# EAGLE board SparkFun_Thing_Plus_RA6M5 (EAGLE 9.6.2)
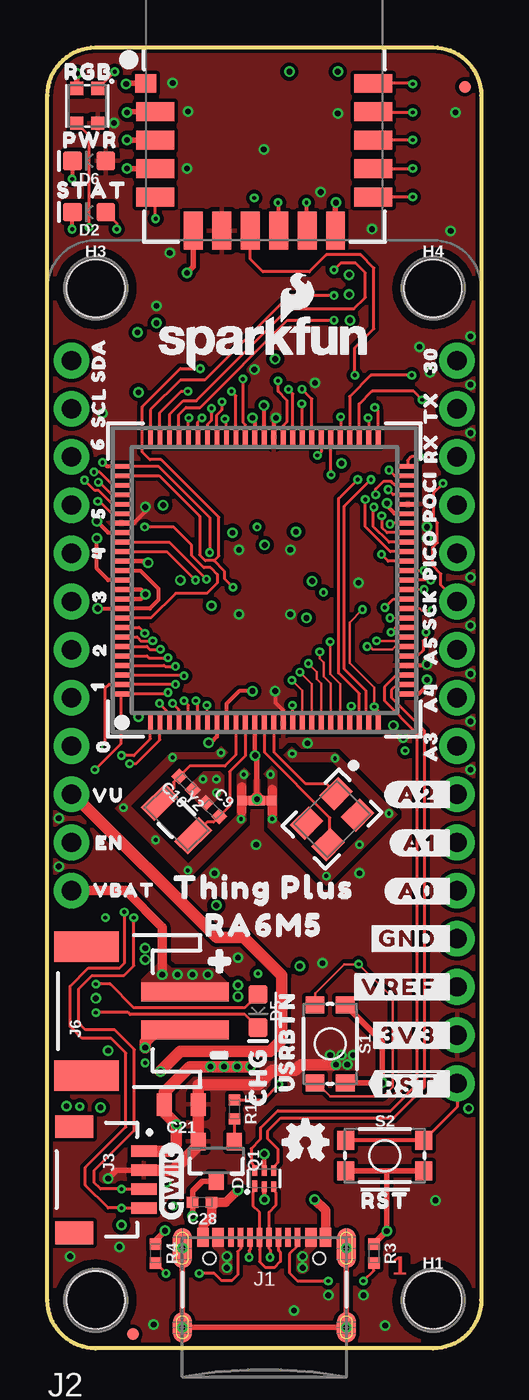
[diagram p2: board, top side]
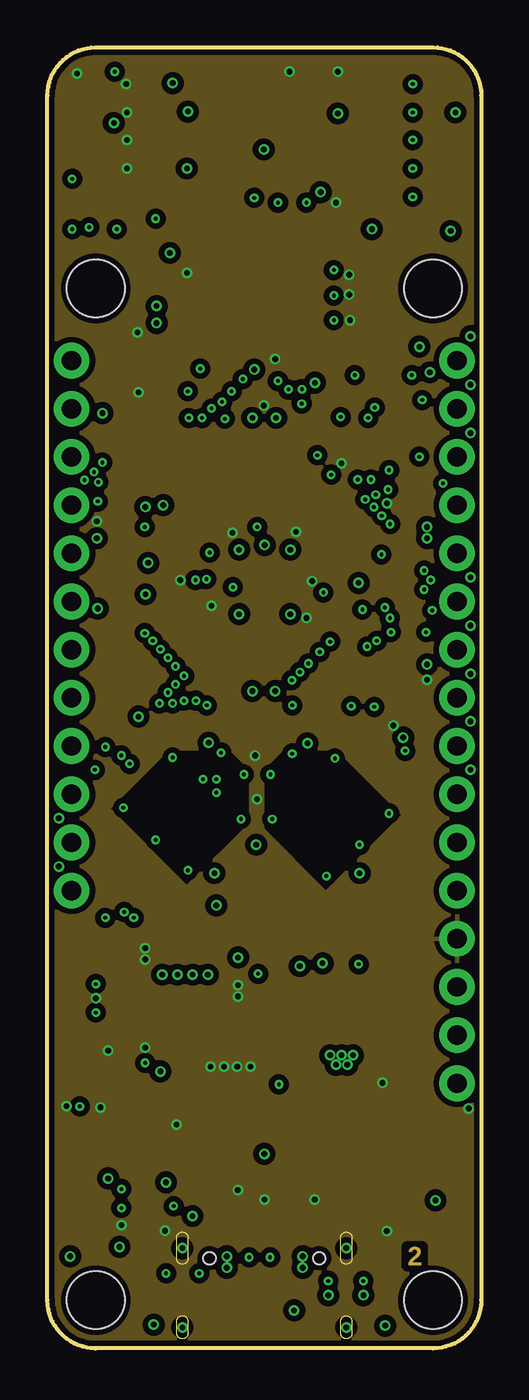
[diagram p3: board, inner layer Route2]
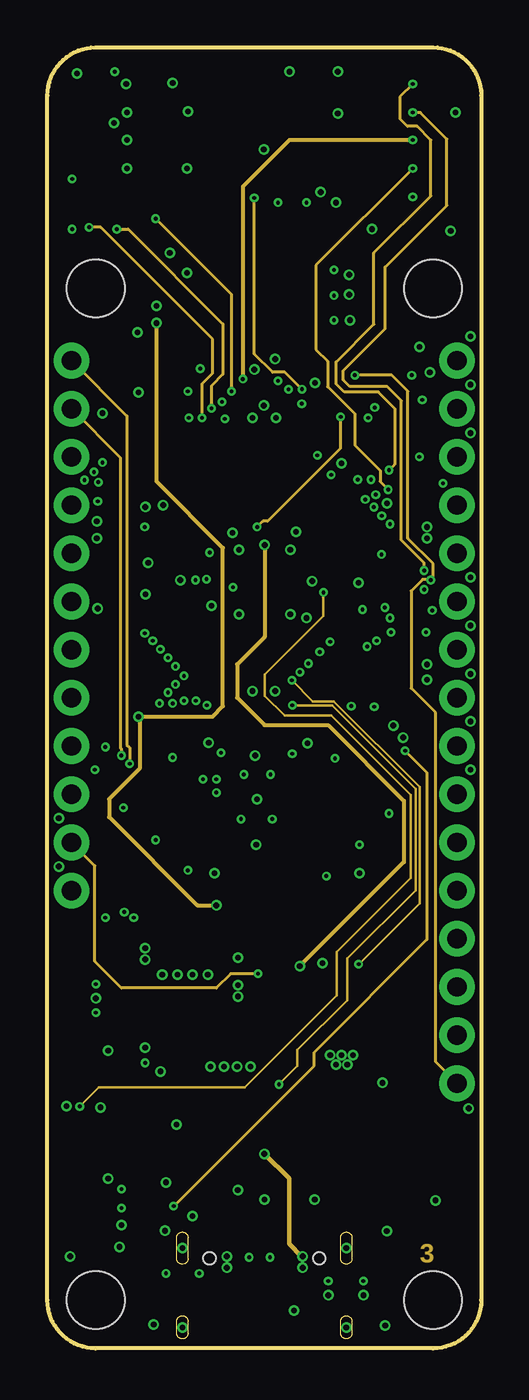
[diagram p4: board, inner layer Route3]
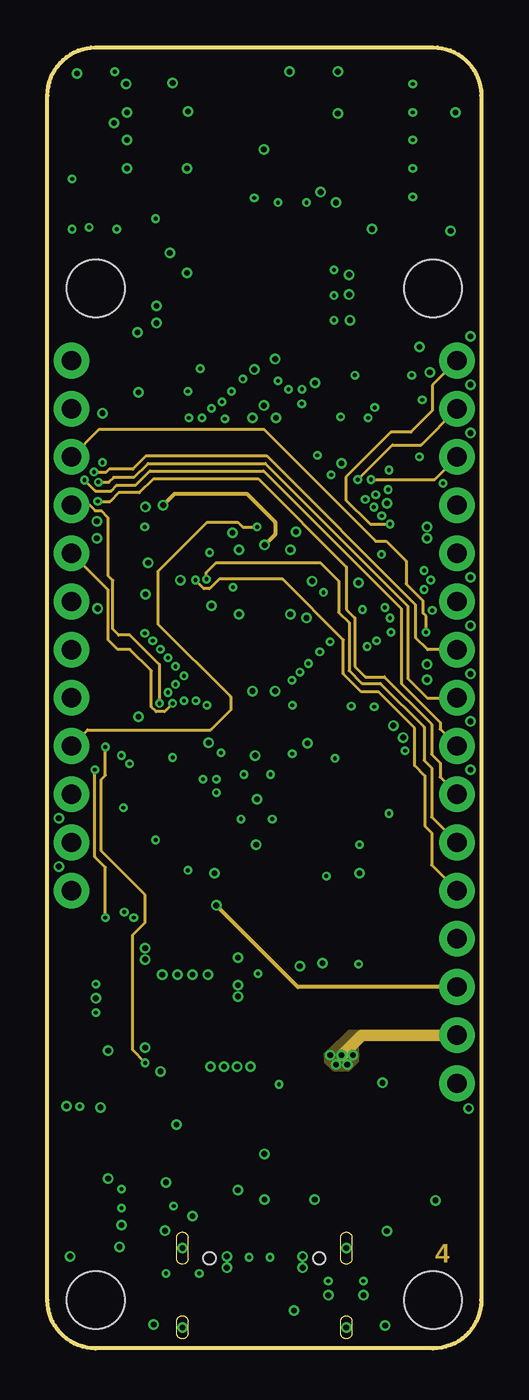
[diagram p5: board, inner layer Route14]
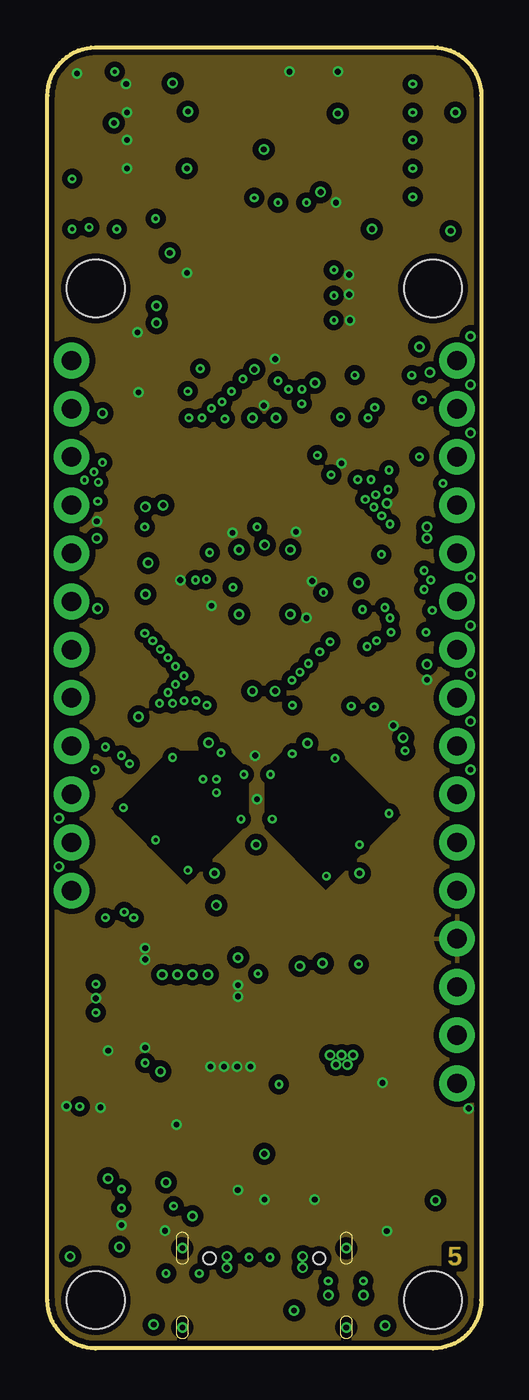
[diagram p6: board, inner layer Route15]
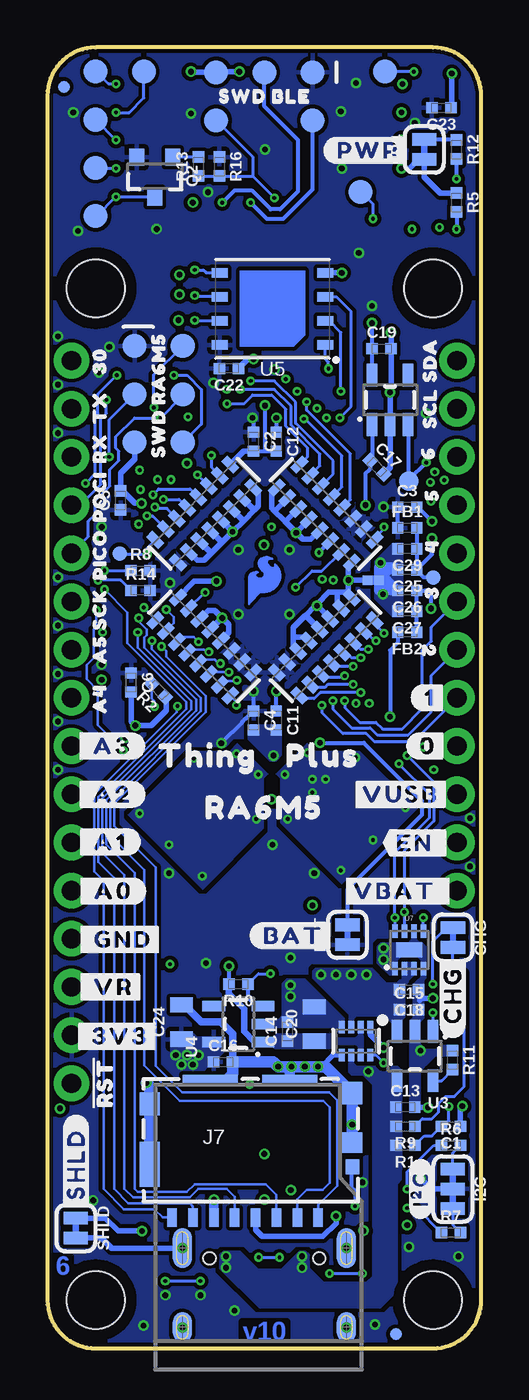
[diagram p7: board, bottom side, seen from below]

Size 22.86 x 68.58 mm. Coordinates in mm from the lower left corner, seen from the top.
Outline: 0,66.04 arc-90 2.54,68.58 20.32,68.58 arc-90 22.86,66.04 22.86,2.54 arc-90 20.32,0 2.54,0 arc-90 0,2.54 0,66.04
Copper layers (1+2*3+14*15+16): Top 0.035mm / dielectric 0.0994mm / Route2 0.0152mm / dielectric 0.55mm / Route3 0.0152mm / dielectric 0.1088mm / Route14 0.0152mm / dielectric 0.55mm / Route15 0.0152mm / dielectric 0.0994mm / Bottom 0.035mm
Design rules "SparkFun-6-Layer-Minimum-JLCPCB": minimum track width 0.09mm, minimum drill 0.2mm, track to track 0.09mm, track to pad 5mil, pad to pad 5mil, via to via 5mil, smd to smd 5mil, copper to edge 7mil, drill to drill 7mil, minimum pad ring 5mil, minimum via ring 5mil, stop-mask expansion 2.5mil, vias tented up to drill 25mil, thermal gap 10mil
Net classes: 2 CLK signals: width 0.15 mm, drill 0.2 mm, clearance 0.15 mm to class 0, clearance 0.15 mm to class 1, clearance 0.15 mm; 3 Analog Ground: width 0.2 mm, clearance 0.2 mm to class 1, clearance 0.3 mm to class 2; 4 Power: width 0.2 mm, drill 0.3 mm, clearance 0.2 mm to class 0, clearance 0.1 mm to class 1, clearance 0.15 mm to class 2, clearance 0.2 mm to class 3, clearance 0.2 mm; 5 USB diff: width 0.16 mm, drill 0.2 mm, clearance 0.3 mm to class 0, clearance 0.3 mm to class 1, clearance 0.3 mm to class 2, clearance 0.3 mm to class 3, clearance 0.2 mm to class 4, clearance 0.22 mm

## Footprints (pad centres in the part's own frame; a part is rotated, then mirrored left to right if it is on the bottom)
SMT-JUMPER_2_NC_TRACE_SILK = smd 0.66 x 1.27: 1 -0.521,0; 2 0.521,0
0402-TIGHT = smd 0.6 x 0.6: 1 -0.5,0; 2 0.5,0
0805 = smd 0.8 x 1.2: 1 -0.9,0; 2 0.9,0
SOT886 = smd 0.61 x 0.25: 1 -0.405,0.5 | smd 0.56 x 0.25: 2 -0.43,0; 3 -0.43,-0.5; 4 0.43,-0.5; 5 0.43,0; 6 0.43,0.5
LED-0603 = smd 1 x 1: A -0.877,0; C 0.877,0
WS2812-2020 = smd 0.7 x 0.7: DI -0.915,0.55; DO 0.915,-0.55; GND 0.915,0.55; VCC -0.915,-0.55
FIDUCIAL-MICRO = smd 0.635 x 0.635: 1 0,0
STAND-OFF-TIGHT = hole 3.048: 0,0
SMT-JUMPER_3_2-NC_TRACE_SILK = smd 0.66 x 1.27: 1 -1.041,0; 2 0,0; 3 1.041,0
USB-C-16P-6LAYER-ISOLATED = smd 0.3 x 1: A5 -1.25,-0.34; A6 -0.25,-0.34; A7 0.25,-0.34; A8 1.25,-0.34; B5 1.75,-0.34; B6 0.75,-0.34; B7 -0.75,-0.34; B8 -1.75,-0.34 | smd 0.6 x 1: GND -3.225,-0.34; GND2 3.225,-0.34; VBUS1 -2.45,-0.34; VBUS2 2.45,-0.34 | smd 1 x 2.1: SHLD1 -4.32,-0.915; SHLD2 4.32,-0.915 | smd 1 x 2.1 bottom: SHLD3 -4.32,-0.915; SHLD4 4.32,-0.915 | smd 1 x 1.6: SHLD5 -4.32,-5.095; SHLD8 4.32,-5.095 | smd 1 x 1.6 bottom: SHLD6 -4.32,-5.095; SHLD7 4.32,-5.095 | hole 0.65: -2.89,-1.445; 2.89,-1.445
THING_PLUS = drill 1.016 pad 1.88: 1 1.27,52.07; 2 1.27,49.53; 3 1.27,46.99; 4 1.27,44.45; 5 1.27,41.91; 6 1.27,39.37; 7 1.27,36.83; 8 1.27,34.29; 9 1.27,31.75; 10 1.27,29.21; 11 1.27,26.67; 12 1.27,24.13; 13 21.59,52.07; 14 21.59,49.53; 15 21.59,46.99; 16 21.59,44.45; 17 21.59,41.91; 18 21.59,39.37; 19 21.59,36.83; 20 21.59,34.29; 21 21.59,31.75; 22 21.59,29.21; 23 21.59,26.67; 24 21.59,24.13; 25 21.59,21.59; 26 21.59,19.05; 27 21.59,16.51; 28 21.59,13.97
JST04_1MM_RA = smd 0.6 x 1.35: 1 -1.5,0; 2 -0.5,0; 3 0.5,0; 4 1.5,0 | smd 1.2 x 2: NC1 2.8,-3.675; NC2 -2.8,-3.675
PAD_05_03X2_TP = smd 1.27 x 1.27: 1 -2.54,-1.27; 2 -2.54,1.27; 3 0,-1.27; 4 0,1.27; 5 2.54,-1.27; 6 2.54,1.27
PAD_05_03X2_TP_NO4 = smd 1.27 x 1.27: 1 -2.54,-1.27; 2 -2.54,1.27; 3 0,-1.27; 5 2.54,-1.27; 6 2.54,1.27
JST-2-SMD = smd 1 x 4.6: 1 -1,-3.7; 2 1,-3.7 | smd 1.6 x 3.4: NC1 -3.4,1.5; NC2 3.4,1.5
MICROSD_TINY = smd 0.5 x 1: 1 3.55,-3.85; 2 2.45,-3.85; 3 1.35,-3.85; 4 0.25,-3.85; 5 -0.85,-3.85; 6 -1.95,-3.85; 7 -3.05,-3.85; 8 -4.15,-3.85 | smd 0.72 x 0.78: 9 5.35,-1.17 | smd 1.05 x 1.08: GND1 5.35,0.1 | smd 1.05 x 1.2: GND2 5.35,2.71; GND3 -5.325,2.14 | smd 1.05 x 2.39: GND4 -5.325,-1.045 | smd 2.91 x 0.55: GND5 -2.145,3.385; GND6 2.045,3.385
SOT23-3 = smd 0.8 x 0.9: 1 -0.95,-1; 2 0.95,-1; 3 0,1.1
2506_AR = smd 0.45 x 0.9: 1 -2.8,-0.85; 2 -2,-0.85; 3 -1.2,-0.85; 4 -0.4,-0.85; 5 0.4,-0.85; 6 1.2,-0.85; 7 2,-0.85; 8 2.8,-0.85; 9 2.8,0.85; 10 2,0.85; 11 1.2,0.85; 12 0.4,0.85; 13 -0.4,0.85; 14 -1.2,0.85; 15 -2,0.85; 16 -2.8,0.85
TACTILE_SWITCH_SMD_4.6X2.8MM = smd 0.9 x 1: 1 -2.05,-0.8; 2 2.05,-0.8; 3 2.05,0.8; 4 -2.05,0.8
2PT_GND_TIE_SMALL = smd 0.5 x 0.5: P$1 0,0.3; P$2 0,-0.3
PAD.03X.05 = smd 1.27 x 1.27: 1 0,0
PAD.03X.04 = smd 1.016 x 1.016: 1 0,0
PAD.03X.03 = smd 0.762 x 0.762: 1 0,0
P-LQFP100-14X14-0.50 = smd 0.25 x 1.1: 1 -6,-7.55; 2 -5.5,-7.55; 3 -5,-7.55; 4 -4.5,-7.55; 5 -4,-7.55; 6 -3.5,-7.55; 7 -3,-7.55; 8 -2.5,-7.55; 9 -2,-7.55; 10 -1.5,-7.55; 11 -1,-7.55; 12 -0.5,-7.55; 13 0,-7.55; 14 0.5,-7.55; 15 1,-7.55; 16 1.5,-7.55; 17 2,-7.55; 18 2.5,-7.55; 19 3,-7.55; 20 3.5,-7.55; 21 4,-7.55; 22 4.5,-7.55; 23 5,-7.55; 24 5.5,-7.55; 25 6,-7.55; 51 6,7.55; 52 5.5,7.55; 53 5,7.55; 54 4.5,7.55; 55 4,7.55; 56 3.5,7.55; 57 3,7.55; 58 2.5,7.55; 59 2,7.55; 60 1.5,7.55; 61 1,7.55; 62 0.5,7.55; 63 0,7.55; 64 -0.5,7.55; 65 -1,7.55; 66 -1.5,7.55; 67 -2,7.55; 68 -2.5,7.55; 69 -3,7.55; 70 -3.5,7.55; 71 -4,7.55; 72 -4.5,7.55; 73 -5,7.55; 74 -5.5,7.55; 75 -6,7.55 | smd 1.1 x 0.25: 26 7.55,-6; 27 7.55,-5.5; 28 7.55,-5; 29 7.55,-4.5; 30 7.55,-4; 31 7.55,-3.5; 32 7.55,-3; 33 7.55,-2.5; 34 7.55,-2; 35 7.55,-1.5; 36 7.55,-1; 37 7.55,-0.5; 38 7.55,0; 39 7.55,0.5; 40 7.55,1; 41 7.55,1.5; 42 7.55,2; 43 7.55,2.5; 44 7.55,3; 45 7.55,3.5; 46 7.55,4; 47 7.55,4.5; 48 7.55,5; 49 7.55,5.5; 50 7.55,6; 76 -7.55,6; 77 -7.55,5.5; 78 -7.55,5; 79 -7.55,4.5; 80 -7.55,4; 81 -7.55,3.5; 82 -7.55,3; 83 -7.55,2.5; 84 -7.55,2; 85 -7.55,1.5; 86 -7.55,1; 87 -7.55,0.5; 88 -7.55,0; 89 -7.55,-0.5; 90 -7.55,-1; 91 -7.55,-1.5; 92 -7.55,-2; 93 -7.55,-2.5; 94 -7.55,-3; 95 -7.55,-3.5; 96 -7.55,-4; 97 -7.55,-4.5; 98 -7.55,-5; 99 -7.55,-5.5; 100 -7.55,-6
DA14531MOD = smd 1.1 x 1: 1 -6.25,1 | smd 2 x 1: 2 -5.75,-0.5; 3 -5.75,-2; 4 -5.75,-3.5; 5 -5.75,-5; 12 5.75,-5; 13 5.75,-3.5; 14 5.75,-2; 15 5.75,-0.5; 16 5.75,1 | smd 1 x 2: 6 -3.75,-6.75; 7 -2.25,-6.75; 8 -0.75,-6.75; 9 0.75,-6.75; 10 2.25,-6.75; 11 3.75,-6.75
SOT23-5 = smd 0.55 x 1.2: 1 -0.95,-1.3; 2 0,-1.3; 3 0.95,-1.3; 4 0.95,1.3; 5 -0.95,1.3
WSON-8-6X5 = smd 0.85 x 0.5: 1 -2.775,1.905; 2 -2.775,0.635; 3 -2.775,-0.635; 4 -2.775,-1.905; 5 2.775,-1.905; 6 2.775,-0.635; 7 2.775,0.635; 8 2.775,1.905
DFN-8 = smd 0.3 x 0.7: 1 -0.75,-0.99; 2 -0.25,-0.99; 3 0.25,-0.99; 4 0.75,-0.99; 5 0.75,0.99; 6 0.25,0.99; 7 -0.25,0.99; 8 -0.75,0.99 | smd 1.38 x 0.8: 9 0,0
SOT8 = smd 0.67 x 0.3: 1 -0.74,0.75; 2 -0.74,0.25; 3 -0.74,-0.25; 4 -0.74,-0.75; 5 0.74,-0.75; 6 0.74,-0.25; 7 0.74,0.25; 8 0.74,0.75
4-SMD,32X25 = smd 1.4 x 1.1: 1 -1.1,-0.8; 2 1.1,-0.8; 3 1.1,0.8; 4 -1.1,0.8
CRYSTAL-SMD-3.2X1.5MM = smd 1 x 1.8: P$1 -1.25,0; P$2 1.25,0

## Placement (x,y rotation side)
BAT  JUMPER-SMT_2_NC_TRACE_SILK  [SMT-JUMPER_2_NC_TRACE_SILK]  7.05,21.8 90 bottom
C1  1.0uF  [0402-TIGHT]  1.6,11.7 180 bottom
C2  0.1uF  [0402-TIGHT]  12,47.8 270 bottom
C3  0.1uF  [0402-TIGHT]  3.9,44.35 0 bottom
C4  0.1uF  [0402-TIGHT]  12,33.1 270 bottom
C5  0.1uF  [0402-TIGHT]  19,44.7 90 bottom
C6  0.1uF  [0402-TIGHT]  18.45,35.1 270 bottom
C9  9.1pF  [0402-TIGHT]  8.7,28.4 315 top
C10  9.1pF  [0402-TIGHT]  7.3,29.8 135 top
C11  0.1uF  [0402-TIGHT]  10.8,33.1 270 bottom
C12  0.1uF  [0402-TIGHT]  10.8,47.8 270 bottom
C13  2.2uF  [0402-TIGHT]  4.01,12.71 0 bottom
C14  2.2uF  [0402-TIGHT]  10.2,16.7 90 bottom
C15  2.2uF  [0402-TIGHT]  3.81,17.86 0 bottom
C16  2.2uF  [0402-TIGHT]  13.6,15.1 0 bottom
C17  2.2uF  [0402-TIGHT]  5.5,46.45 315 bottom
C18  0.1uF  [0402-TIGHT]  3.8,18.9 180 bottom
C19  1.0uF  [0402-TIGHT]  5.25,52.7 0 bottom
C20  10uF  [0805]  8.8,17.1 90 bottom
C21  10uF  [0805]  7.05,12.85 180 top
C22  0.1uF  [0402-TIGHT]  13.3,51.65 180 bottom
C23  0.1uF  [0402-TIGHT]  2.1,65.4 180 bottom
C24  47uF/6.3V  [0805]  15.8,17.2 90 bottom
C25  0.1uF  [0402-TIGHT]  3.9,41.05 180 bottom
C26  0.1uF  [0402-TIGHT]  3.9,39.95 180 bottom
C27  1.0uF  [0402-TIGHT]  3.9,38.85 180 bottom
C28  0.1uF  [0402-TIGHT]  8.15,7.7 180 top
C29  1.0uF  [0402-TIGHT]  3.9,42.15 180 bottom
CHG  JUMPER-SMT_2_NC_TRACE_SILK  [SMT-JUMPER_2_NC_TRACE_SILK]  1.49,21.66 270 bottom
D1  PRTR5V0U2F  [SOT886]  11.43,8.95 90 top
D2  BLUE  [LED-0603]  2.2,59.9 180 top
D4  WS2812_2020  [WS2812-2020]  2.1,65.5 90 top
D5  Yellow  [LED-0603]  11.1,17.78 270 top
D6  [LED-0603]  2.2,62.6 180 top
FB1  120-OHM  [0402-TIGHT]  3.9,43.25 0 bottom
FB2  120-OHM  [0402-TIGHT]  3.9,37.75 180 bottom
FD1  FIDUCIALUFIDUCIAL  [FIDUCIAL-MICRO]  22,66.5 0 top
FD2  FIDUCIALUFIDUCIAL  [FIDUCIAL-MICRO]  4.5,0.75 0 bottom
FD3  FIDUCIALUFIDUCIAL  [FIDUCIAL-MICRO]  22,66.5 0 bottom
FD4  FIDUCIALUFIDUCIAL  [FIDUCIAL-MICRO]  4.5,0.75 0 top
FRAME1  FRAME-LEDGER  [CREATIVE_COMMONS]  not placed on the board
FRAME2  FRAME-LEDGERNO_FOOTPRINT  [DUMMY]  24.28,1.89 0 top
H1  STAND-OFFTIGHT  [STAND-OFF-TIGHT]  20.32,2.54 0 top
H2  STAND-OFFTIGHT  [STAND-OFF-TIGHT]  2.54,2.54 0 top
H3  STAND-OFFTIGHT  [STAND-OFF-TIGHT]  2.54,55.88 0 top
H4  STAND-OFFTIGHT  [STAND-OFF-TIGHT]  20.32,55.88 0 top
I2C  JUMPER-SMT_3_2-NC_TRACE_SILK  [SMT-JUMPER_3_2-NC_TRACE_SILK]  1.5,8.4 270 bottom
J1  USB Female Type C Connector  [USB-C-16P-6LAYER-ISOLATED]  11.43,6.2 0 top
J2  THING_PLUS_LOGICAL  [THING_PLUS]  0,0 0 top
J3  QWIIC_RA  [JST04_1MM_RA]  5.08,8.89 270 top
J4  CONN_03X2  [PAD_05_03X2_TP]  17,50.3 270 bottom
J5  [PAD_05_03X2_TP_NO4]  11.43,66 180 bottom
J6  [JST-2-SMD]  3.56,17.78 90 top
J7  MICRO-SDFRICTION  [MICROSD_TINY]  12.14,10.74 0 bottom
JP4  JUMPER-SMT_2_NC_TRACE_SILK  [SMT-JUMPER_2_NC_TRACE_SILK]  3,63.2 90 bottom
LOGO1  OSHW-LOGOMINI  [OSHW-LOGO-MINI]  13.6,10.88 0 top
LOGO2  SFE_LOGO_NAME_FLAME.1_INCH  [SFE_LOGO_NAME_FLAME_.1]  11.43,53 0 top
LOGO3  QWIIC_LOGO_4MM  [QWIIC_4MM]  6.54,8.82 90 top
LOGO4  SFE_LOGO_NAME_FLAMEBLANK  [BLANK]  23.26,0.88 0 top
Q1  20V/4.2A/52mΩ/1.4W  [SOT23-3]  8.9,9.9 180 top
Q2  20V/4.2A/52mΩ/1.4W  [SOT23-3]  17.2,61.8 180 bottom
R1  1k  [0402-TIGHT]  4,10.7 180 bottom
R2  20k  [0402-TIGHT]  17,34.7 135 bottom
R3  5.1k  [0402-TIGHT]  17.2,5 270 top
R4  5.1k  [0402-TIGHT]  5.7,5 270 top
R5  2.2k  [0402-TIGHT]  1.3,60.4 270 bottom
R6  2.2k  [0402-TIGHT]  1.6,10.7 0 bottom
R7  2.2k  [0402-TIGHT]  1.6,6.1 0 bottom
R8  10k  [0402-TIGHT]  17.95,41 0 bottom
R9  4.7k  [0402-TIGHT]  4,11.7 180 bottom
R10  1M  [0402-TIGHT]  12.8,19.2 180 bottom
R11  4.7k  [0402-TIGHT]  1.52,15.19 270 bottom
R12  4.7k  [0402-TIGHT]  1.3,63.2 270 bottom
R13  1k  [0402-TIGHT]  14.9,62.3 90 bottom
R14  10k  [0402-TIGHT]  17.95,39.95 0 bottom
R15  1k  [0402-TIGHT]  9.85,12.6 270 top
R16  10k  [0402-TIGHT]  13.8,62.3 270 bottom
RN1  10K  [2506_AR]  8.2,44 315 bottom
RN3  10K  [2506_AR]  14.6,37 135 bottom
RN4  10K  [2506_AR]  14.6,44 45 bottom
RN5  10K  [2506_AR]  8.2,37 45 bottom
S1  USER  [TACTILE_SWITCH_SMD_4.6X2.8MM]  14.9,16.05 270 top
S2  RESET  [TACTILE_SWITCH_SMD_4.6X2.8MM]  17.78,10.16 0 top
SHLD  JUMPER-SMT_2_NC_TRACE_SILK  [SMT-JUMPER_2_NC_TRACE_SILK]  21.36,6.34 270 bottom
SUPPLYTIE1  2PT_GND_TIESMALL  [2PT_GND_TIE_SMALL]  5.7,40.5 270 bottom
SUPPLYTIE2  2PT_GND_TIESMALL  [2PT_GND_TIE_SMALL]  10.56,28.87 90 top
SUPPLYTIE3  2PT_GND_TIESMALL  [2PT_GND_TIE_SMALL]  11.5,28.87 90 top
TP1  TEST-POINT3X5  [PAD.03X.05]  5.08,67.31 0 bottom
TP2  TEST-POINT3X4  [PAD.03X.04]  3.81,45.72 90 bottom
TP3  TEST-POINT3X5  [PAD.03X.05]  20.32,59.69 0 bottom
TP4  TEST-POINT3  [PAD.03X.03]  2.54,40.64 0 bottom
TP5  TEST-POINT3X5  [PAD.03X.05]  20.32,64.77 0 bottom
TP6  TEST-POINT3X5  [PAD.03X.05]  6.35,60.96 0 bottom
TP7  TEST-POINT3X5  [PAD.03X.05]  20.32,62.23 0 bottom
TP8  TEST-POINT3X5  [PAD.03X.05]  20.32,67.31 0 bottom
TP9  TEST-POINT3  [PAD.03X.03]  19.05,41.91 0 bottom
TP10  TEST-POINT3X5  [PAD.03X.05]  17.78,67.31 0 bottom
U1  R7FA6M5  [P-LQFP100-14X14-0.50]  11.43,40.5 0 top
U2  DA14531MOD  [DA14531MOD]  11.43,65.68 0 top
U3  MCP73831  [SOT23-5]  3.5,15.41 180 bottom
U4  RT9080-33GJ5  [SOT23-5]  12.8,17.1 90 bottom
U5  MX25L12833F 128Mb  [WSON-8-6X5]  11,54.8 180 bottom
U6  RT9080-33GJ5  [SOT23-5]  4.8,50 0 bottom
U7  MAX17048  [DFN-8]  3.8,21 0 bottom
U8  LM66200  [SOT8]  6.6,16.2 270 bottom
U$3  [#I�C#0]  3.2,8.4 90 bottom
U$4  [#CHG#0]  1.5,18.6 90 bottom
U$8  [SFE_LOGO_FLAME_COPPER_EXPOSED_.1]  11.43,40.5 0 bottom
U$9  [SWD_RA6M50]  17,50.25 90 bottom
U$10  [SWD_BLE0]  11.4,66 0 bottom
U$12  [300]  20.2,52.1 90 top
U$13  [#RST#0]  17.8,7.9 0 top
U$14  [CHG0]  11.1,14.3 90 top
U$15  [STAT0]  2.35,61.05 0 top
U$16  [PWR0]  2.25,63.7 0 top
U$17  [RGB0]  2.15,67.3 0 top
U$18  [THING_PLUS0]  11.43,24.3 0 top
U$19  [##RST#_#0]  21.55,13.95 0 top
U$20  [#3V3_#0]  21.55,16.5 0 top
U$21  [#VREF_#0]  21.55,19.05 0 top
U$22  [#GND_#0]  21.55,21.6 0 top
U$23  [#A0_#0]  21.55,24.1 0 top
U$24  [#A1_#0]  21.55,26.65 0 top
U$25  [#A2_#0]  21.55,29.2 0 top
U$26  [A30]  20.2,31.75 90 top
U$27  [A40]  20.2,34.3 90 top
U$28  [A50]  20.2,36.8 90 top
U$29  [SCK0]  20.15,38.95 90 top
U$30  [PICO0]  20.15,41.85 90 top
U$31  [POCI0]  20.15,44.9 90 top
U$32  [RX0]  20.2,47.45 90 top
U$33  [TX0]  20.2,49.6 90 top
U$34  [60]  2.65,47.7 90 top
U$35  [SDA0]  2.7,52.1 90 top
U$36  [SCL0]  2.7,49.6 90 top
U$37  [50]  2.7,44.05 90 top
U$38  [40]  2.7,41.95 90 top
U$39  [30]  2.75,39.65 90 top
U$40  [20]  2.75,36.85 90 top
U$41  [10]  2.65,34.9 90 top
U$42  [00]  2.95,31.75 90 top
U$43  [60]  2.8,47.2 90 bottom
U$44  [VU0]  3.2,29.15 0 top
U$45  [EN0]  3.25,26.65 0 top
U$46  [VBAT0]  4.05,24.15 0 top
U$47  [#PWR#0]  5.95,63.15 0 bottom
U$48  [50]  2.6,45 90 bottom
U$49  [#BAT#0]  9.9,21.75 0 bottom
U$50  [#SHLD#0]  21.35,9.7 90 bottom
U$51  [#RST#0]  19.95,14 90 bottom
U$52  [#_3V3#0]  19.2,16.45 0 bottom
U$53  [#_VR#0]  21.45,19.05 0 bottom
U$54  [#_GND#0]  19.05,21.55 0 bottom
U$55  [#_A0#0]  19.55,24.1 0 bottom
U$56  [#_A1#0]  19.7,26.7 0 bottom
U$57  [#_A2#0]  19.6,29.2 0 bottom
U$58  [#_A3#0]  19.6,31.75 0 bottom
U$59  [A40]  20.1,34.25 90 bottom
U$60  [A50]  20.1,36.85 90 bottom
U$61  [SCK0]  20.1,38.95 90 bottom
U$62  [PICO0]  20.1,41.85 90 bottom
U$63  [POCI0]  20.1,44.9 90 bottom
U$64  [RX0]  20.1,47.45 90 bottom
U$65  [TX0]  20.1,49.6 90 bottom
U$66  [40]  2.6,42.3 90 bottom
U$67  [SDA0]  2.7,52.1 90 bottom
U$68  [SCL0]  2.7,49.55 90 bottom
U$69  [30]  2.6,39.85 90 bottom
U$70  [20]  2.75,36.75 270 bottom
U$71  [#1#0]  2.7,34.3 0 bottom
U$72  [#0#0]  2.8,31.75 0 bottom
U$73  [#USRBTN#0]  12.5,16.15 90 top
U$76  [#VUSB#0]  4.25,29.2 0 bottom
U$77  [#EN_#0]  3.35,26.65 0 bottom
U$78  [#VBAT_#0]  4.4,24.1 0 bottom
U$79  [RA6M50]  11.43,22.3 0 top
U$80  [ORDERING_INSTRUCTIONS]  not placed on the board
U$81  [#0]  9.2,20.4 0 top
U$82  [RA6M50]  11.43,28.5 0 bottom
U$83  [THING0]  14.4,31.25 0 bottom
U$84  [PLUS0]  8.35,31.25 0 bottom
U$85  [_#0]  8.85,15.45 0 top
U$86  [300]  20.1,52.05 90 bottom
Y1  24.000MHz  [4-SMD,32X25]  15,27.9 225 top
Y2  32.768kHz  [CRYSTAL-SMD-3.2X1.5MM]  6.8,27.9 315 top

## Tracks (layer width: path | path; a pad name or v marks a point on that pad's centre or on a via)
3.3V  (via drill 0.3)
  Top 0.2: 11.93,48.95 U1.62 | v20,36.05 19.95,36 U1.29 | U1.82 4.55,43.5 5.16,44.11 v5.16,44.35 | U1.15 12.43,33.63 12.03,34.03 12.03,34.62 v12,34.65
  Top 0.3: J3.2 3.64,9.39 v3.2,8.95
  Top 0.6: J3.2 6.64,9.39 7.95,10.7 Q1.2 C21.1 7.95,13.9 11.1,13.9 11.85,14.65 13.05,14.65 13.35,14.95 v15.2,14.95
  Route14 0.6: J2.27 16.56,16.51 v15.5,15.45
  Bottom 0.2: v12,34.65 C4.1 12.4,33.2 12.42,33.2 12.6,33.02 12.6,33 v13.7,31.9 | C2.1 12,49.02 | FB1.1 C3.1
  Bottom 0.3: v3.2,8.95 2.65,8.4 I2C.2
  other vias: 14.9,15.45 16.1,15.45 15.8,14.95 3.5,64.6 12.05,49.05 20,43.3 10.1,42.1 12.8,42.1 12.8,38.7 10.1,38.7 16.4,40.35 18.75,32.2 14.1,50.9 19.6,52.8 11,26.55 16.45,25.05 8.8,25.05 14.5,20.3 10.9,51.6 5.75,54.95 7.4,65.2 6.6,66.7 7.35,62.2 15.3,65.1 11.4,63.2 14.4,60.95 17.1,59 21.25,58.9 21.5,65.15 6.45,57.75 13,2 14.8,2.8 16.65,2.8 5.6,1.25 3.8,5.35 1.2,4.85 17.8,1.2 6.25,8.75 20.45,7.8 22.3,33.05 22.3,30.5 22.3,35.55 22.3,38.1 22.3,40.65 20,42.7 22.3,48.25 22.3,50.8 20.15,51.45 22.3,53.35 2.9,49.3 0.6,25.4 0.6,27.95 10.05,20.6
  pour Bottom (isolate 0.15, rank 2, no thermals): 13.8,14.85 13.85,14.8 14.4,14.8 14.6,14.6 16,14.6 16.4,15 16.4,16.6 16.35,16.65 15.2,16.65 15,16.45 13.55,16.45 13.5,16.4 13.5,15.65 13.8,15.35
  pour Top (isolate 0.2, rank 3): 0,0 22.85,0 22.85,68.6 0,68.6
  pour Bottom (isolate 0.2, rank 3): 0,0 22.85,0 22.85,68.6 0,68.6
  pour Route14 (no thermals): 16.65,16.8 15.85,16.8 14.7,15.65 14.6,15.55 14.6,15.3 14.6,15.05 15,14.65 15.05,14.6 15.9,14.6 16.4,15.1 16.4,15.3 16.4,15.95 16.65,16.2
  pour Top: 16.4,59.75 16.3,59.75 15.9,60.15 15.9,60.25 15.75,60.25 16,60 16,59.85 16.25,59.6
  pour Top: 6.6,59.85 6.75,59.85 6.95,60.05 6.95,60.25 7.15,60.25 7.15,60.15 6.8,59.8 6.65,59.8
3.3V_SW  (via drill 0.3)
  Top 0.3: v7.65,6.97 C28.2 7.65,8.3 8.15,8.8 Q1.3
  Bottom 0.3: J7.4 11.89,6.24 11.54,5.89 8.35,5.89 7.65,6.59 v7.65,6.97
!CTS_RA6/RTS_DA14531!  (via drill 0.2)
  Top 0.15: U2.13 19.23,62.18 v19.25,62.2 | U1.47 18.22,45 v17.95,45.27
  Route3 0.15: v19.25,62.2 14.15,57.1 14.15,52.65 14.77,52.03 14.77,50.69 16.2,49.26 16.2,47.61 17.53,46.28 17.53,45.69 v17.95,45.27
  Bottom 0.15: v19.25,62.2 20.29,62.2 TP7.1
!DA14531_RST!  (via drill 0.2)
  Top 0.15: U1.58 13.93,50.04 v13.41,50.56
  Route3 0.15: v13.41,50.56 12.51,51.46 11.86,51.46 10.9,52.42 v10.9,60.65
  Bottom 0.15: J5.6 12.05,62.81 12.05,61.8 | R13.1 R16.2 12.05,61.8 | 12.05,61.8 v10.9,60.65
!FG_ALRT!  (via drill 0.2)
  Top 0.15: v6.35,34.57 6.28,34.5 U1.100 3.88,31.88 v2.5,30.5
  Route14 0.15: v3.05,22.7 3.05,25.36 2.5,25.91 v2.5,30.5
  Bottom 0.15: U7.5 v3.05,22.7 | RN5.1 9.41,34.25 8.8,34.25 8.48,34.57 v6.35,34.57
!NMI!  (via drill 0.2)
  Top 0.15: U1.40 17.95,41.5 v17.6,41.85
  Bottom 0.15: RN4.16 17.6,42.2 v17.6,41.85 v17.61,41.86 19,41.86 TP9.1
!QCS!  (via drill 0.2)
  Top 0.15: U1.77 5.89,46 8.02,43.87 8.02,41.82 8.32,41.52 8.78,41.52 | v8.05,51.65 7.01,51.65 5,49.64 5,47.25 5.4,46.85 6,46.85 9.03,43.82 9.03,41.77 8.78,41.52 | v9.78,40.12 9.33,40.57 9.33,40.97 8.78,41.52
  Bottom 0.15: RN1.7 8.39,40.98 8.91,40.98 9.77,40.12 v9.78,40.12 | v8.05,51.65 8.05,52 8.22,52.17 U5.1
!RA6M5_RESET!  (via drill 0.2)
  Top 0.15: v20.2,40.5 U1.38 | v16.2,51.3 16.2,52.75 17.2,53.75 17.2,56.95 16.5,57.65 14.7,57.65 13.8,56.75 11.35,56.75 10.68,57.42 U2.8 | J2.28 21.59,12.72 S2.3
  Top 0.2: S2.3 S2.4
  Route3 0.15: J2.28 20.45,15.11 20.45,33.52 19.17,34.8 19.17,39.93 19.77,40.53 20.17,40.53 v20.2,40.5 20.26,40.5 20.33,40.57 20.33,41.37 19,42.7 19,50.45 18.15,51.3 v16.2,51.3
  Bottom 0.15: R14.1 19,40.5 v20.2,40.5 | v16.2,51.3 15.5,51.3 14.74,50.55 14.74,48.72 15.71,47.76 J4.6
!RTS_RA6/CTS_DA14531!  (via drill 0.2)
  Top 0.15: v19.25,66.65 19.22,66.68 U2.16 | U1.49 18.3,46 v18,46.3
  Route3 0.15: v19.25,66.65 18.57,65.97 18.57,64.82 18.97,64.42 19.48,64.42 20.2,63.7 20.2,60.75 17.2,57.75 17.2,53.99 15.21,52 15.21,50.84 15.64,50.41 17.44,50.41 18.3,49.55 18.3,46.6 v18,46.3
  Bottom 0.15: TP8.1 19.67,66.67 19.27,66.67 v19.25,66.65
!SD_EN!  (via drill 0.2)
  Top 0.15: R15.1 11.39,13.1 v12.2,13.91 | U1.16 12.93,33.88 v12.91,33.9
  Route3 0.12: v12.91,33.9 15,33.9 19.4,29.5 19.4,24.15 15.8,20.55 15.8,18.35 13.18,15.72 13.18,14.89 v12.2,13.91
  Bottom 0.15: v12.91,33.9 12.91,34.1 RN3.16
!USR_BTN!  (via drill 0.2)
  Top 0.12: U1.17 13.43,34.67 v12.88,35.22 | S1.1 14.1,18.7 15.65,20.25 v16.4,20.25 16.42,20.25 18.19,18.48 18.19,13.78 17.7,13.29 14.89,13.29 14.18,14 S1.2
  Route3 0.12: v12.88,35.22 13.99,34.11 15.09,34.11 19.61,29.59 19.61,23.46 v16.4,20.25
  Bottom 0.12: v12.88,35.22 12.93,35.17 13.6,35.17 RN3.15
A0/DAC0/D7  (via drill 0.2)
  Top 0.15: U1.85 6.3,42 v7.8,40.5
  Route14 0.15: J2.24 20.24,25.48 20.24,27.18 19.89,27.53 19.89,30.18 19.35,30.72 19.35,32.7 17.45,34.6 16.55,34.6 15.6,35.55 15.6,37.35 12.4,40.55 9.05,40.55 8.55,40.05 8.25,40.05 v7.8,40.5
A1/DAC1/D8  (via drill 0.2)
  Top 0.15: U1.84 6.41,42.5 8.36,40.55 v8.38,40.55
  Route14 0.15: v8.38,40.55 8.38,40.9 8.88,41.4 14.4,41.4 15.35,40.45 15.35,38.8 15.9,38.25 15.9,35.73 16.57,35.05 17.55,35.05 19.85,32.75 19.85,31 20.25,30.6 20.25,28.01 J2.23
A2/D9  (via drill 0.2)
  Top 0.15: U1.81 3.4,44 2.75,44.65 v2.65,44.65
  Route14 0.15: v2.65,44.65 3.3,44.65 3.75,45.1 4.85,45.1 5.6,45.85 11.1,45.85 15.75,41.2 15.75,38.95 16.2,38.5 16.2,35.95 16.75,35.4 17.75,35.4 20.24,32.91 20.24,31.31 20.69,30.86 20.69,30.11 J2.22
A3/D10  (via drill 0.2)
  Top 0.15: U1.80 3.42,44.5 2.7,45.22 2.5,45.22 v1.95,45.77
  Route14 0.15: v1.95,45.77 2.52,45.2 3.35,45.2 3.65,45.5 4.65,45.5 5.4,46.25 11.39,46.25 18.65,38.99 18.65,35.04 20.69,33 20.69,32.65 J2.21
A4/D11  (via drill 0.2)
  Top 0.15: U1.79 3.39,45 2.73,45.66 v2.68,45.66
  Route14 0.15: v2.68,45.66 3.23,45.66 3.48,45.91 4.56,45.91 5.3,46.65 11.48,46.65 19,39.13 19,35.3 20.01,34.29 J2.20
A5/D12  (via drill 0.2)
  Top 0.15: U1.78 3.45,45.5 2.75,46.2 v2.45,46.2
  Route14 0.15: v2.45,46.2 3.1,46.2 3.25,46.35 4.5,46.35 5.2,47.05 11.55,47.05 19.39,39.21 19.39,37.48 20.04,36.83 J2.19
AGND  (via drill 0.3)
  Top 0.25: U1.89 4.92,40 v5.17,39.75 v5.17,39.74 4.93,39.5 U1.90 | U1.86 5.22,41.5 v5.31,41.41
  Bottom 0.5: SUPPLYTIE1.P$1 5.4,39.95 5.05,39.95 | 5.05,39.95 C26.2 4.95,40.5 SUPPLYTIE1.P$1 | SUPPLYTIE1.P$1 5.4,41.15 5.35,41.2 4.55,41.2 C25.2 4.85,41.05 SUPPLYTIE1.P$1 | SUPPLYTIE1.P$1 5.05,40.15 5.05,39.95
  pour Bottom (no thermals): 4.1,38.6 4.15,38.55 4.7,38.55 5.65,39.5 5.65,41.5 4.7,42.45 4.15,42.45 4.1,42.4
AVCC0  (via drill 0.3)
  Top 0.2: U1.88 3.2,40.5 2.6,41.1 v2.6,42.7
  Bottom 0.2: FB1.2 C29.1 C25.1 | C25.1 2.6,41.85 v2.6,42.7 | TP4.1 3.04,40.64 3.4,41 C25.1
BAT_SW  (via drill 0.2)
  Top 0.15: v6.75,35 U1.99 3.25,35 3.05,34.8 v3.05,31.7
  Route14 0.15: v5.15,15.05 v5.16,15.06 4.5,15.72 4.5,21.8 5.15,22.45 5.15,23.9 2.84,26.21 2.84,30 3.05,30.21 v3.05,31.7
  Bottom 0.15: U8.8 5.56,15.46 v5.15,15.05 | RN5.2 8.88,34.85 8.23,34.85 8.08,35 v6.75,35
BLE_RST  (via drill 0.2)
  Top 0.15: v19.25,60.7 19.23,60.68 U2.12
  Bottom 0.15: TP3.1 20.27,59.69 v19.26,60.7 v19.25,60.7 Q2.3
BOOT/MD  (via drill 0.2)
  Top 0.15: U1.39 v19.85,41 | v19.25,65.15 17.21,65.15 U2.15
  Route3 0.15: v19.85,41 19.85,41.4 18.65,42.6 18.65,49.95 17.9,50.7 15.94,50.7 15.6,51.04 15.6,51.55 17.8,53.75 17.8,57 21.05,60.25 21.05,63.75 19.65,65.15 v19.25,65.15
  Bottom 0.15: v19.85,41 R8.1 | v19.25,65.15 18.55,65.15 17.78,65.92 TP10.1
DA14531_SWCLK  (via drill 0.2)
  Top 0.2: U2.10 13.65,58.96 v13.65,60.4
  Bottom 0.2: v13.65,60.4 13,61.05 12.1,61.05 11.1,60.05 10.6,60.05 9.65,61 9.65,63.7 11.43,65.48 J5.3
DA14531_SWDIO  (via drill 0.2)
  Top 0.2: U2.9 12.18,60.37 v12.15,60.4
  Bottom 0.2: v12.15,60.4 11.3,59.55 10.44,59.55 8.89,61.1 J5.2
EXTAL
  Top 0.15: U1.14 11.93,31.43 13.59,29.77 14.69,29.77 Y1.1
FREE/D30  (via drill 0.2)
  Top 0.15: U1.44 18.1,43.5 v18.05,43.45
  Route14 0.15: J2.13 20.29,50.77 20.29,49.44 19.15,48.3 18.1,48.3 15.73,45.93 15.73,44.73 17,43.45 v18.05,43.45
GND  (via drill 0.3)
  Top 0.2: v2.6,43.6 3.2,43 U1.83 | v17.9,44.55 17.9,44.4 18.3,44 U1.45 | v11.4,49.7 11.43,49.67 U1.63 | v20,35.25 20,34.92 19.58,34.5 U1.26
  Top 0.25: D1.2 v11.43,7.84 | U1.12 10.93,31.27
  Top 0.3: v6.2,6.2 5.7,5.7 R4.1 | S2.1 17.9,9.36 | 17.9,9.36 S2.2 | R3.1 v17.88,6.18 v17.88,6.19 17.88,9.34 17.9,9.36 | v1.55,67.2 D4.GND | U2.1 4.18,66.68 v4.15,66.65 | U2.2 4.23,65.18 v4.2,65.15 | U2.3 4.22,63.68 v4.2,63.7 | U2.4 4.22,62.18 v4.2,62.2 | U2.6 7.68,57.03 v7.35,56.7 | U2.11 15.18,60.38 v15.2,60.4 | 11.03,29.37 11.03,31.17 v10.95,31.25 10.93,31.27 | SUPPLYTIE2.P$2 10.94,28.95 v11.05,28.95 | S1.3 v17.65,14 17.65,16.15 S1.4
  Top 0.5: 11,29.11 10.86,28.97 SUPPLYTIE2.P$2 SUPPLYTIE3.P$1 11.2,28.97 11.07,29.1 | J1.GND 8.21,6.5 8.65,6.94 C28.1 9.4,7.7 v10.03,8.34 | J1.GND2 14.65,7.26 v14.08,7.84
  Top 0.6: J3.1 6.44,10.39 6.8,10.75 v6.8,11.8 6.15,12.45 C21.2 | C21.2 6.15,12.75 | C21.2 6.15,13.5 7.5,14.85 v8.6,14.85 v9.3,14.85 v10,14.85 v10.7,14.85 | v5.15,15.85 5.15,16.15 5.78,16.78 J6.1
  Bottom 0.2: v2.6,43.6 3.35,44.35 C3.2 | v11.4,49.7 11.4,47.3 | 11.4,47.3 C12.2 | C2.2 11.4,47.3 | 13.94,67.3 J5.5
  Bottom 0.3: C13.2 3.49,12.7 v2.8,12.7 | C1.1 1.1,12.67 v1,12.77 | v2.55,18.45 3.15,18.45 3.25,18.35 | v14.08,7.84 14.09,7.83 | SHLD.1 19.81,6.86 19.14,6.19 v17.88,6.19 | v5.15,15.85 5.85,16.55 U8.1 | U8.5 7.79,15.46 8.4,14.85 v8.6,14.85 | SUPPLYTIE1.P$2 v7,40.5 | v7,40.5 7,41.24 RN1.8 | v7,40.5 7,39.76 RN5.9 7.11,39.87 7.6,39.87 | v17.9,44.55 18.25,44.55 18.9,45.2 C5.2 19,46.15 18.27,46.88 J4.5 | C6.2 18.45,33.05 v18.23,32.83 18.21,32.84 17.38,32.84 16.6,33.63 16.6,34.3 R2.1 | RN3.5 13.67,38.5 v13.65,38.5 | RN3.8 15.11,40.45 v13.95,40.45 | RN1.5 8.98,42.65 9.4,42.65 v9.75,43 | RN1.4 9.75,43.02 v9.75,43 | R5.1 2.15,60.9 3,61.75 JP4.1 3.32,62.68 3.8,62.2 v4.2,62.2 | C23.1 1.55,65.45 v1.55,67.2 | v7.35,56.7 v7.36,56.7 U5.4 | v9.75,43 10.35,43.6 | 10.35,43.6 10.95,44.2 | 10.95,44.2 11.05,44.3 11.05,45.11 RN1.1 | RN1.2 10.83,44.2 10.95,44.2 | RN1.3 10.3,43.6 10.35,43.6 | 12.4,44.63 RN4.7 11.97,44.2 11.95,44.2 | RN4.5 13.1,43.07 | 13.1,43.07 v13.1,43.05 13.65,42.5 | 12.5,43.65 13.08,43.07 13.1,43.07 | RN4.6 12.55,43.65 12.5,43.65 | 14.22,41.92 14.6,41.55 14.98,41.55 RN4.2 | 14.22,41.92 13.65,42.5 | RN4.3 14.22,41.93 14.22,41.92 | RN3.6 14.4,38.9 14.05,38.9 v13.65,38.5 | v13.65,38.5 13.3,38.15 13.3,37.73 RN3.4 | J5.5 15.27,67.27 v15.3,67.3 | RN4.4 13.67,42.5 13.65,42.5 | C22.1 12.3,52.15 v12,52.15 | RN5.14 9.9,37 9.9,37.5 | 7.6,39.87 8.03,39.87 8.65,39.25 v8.65,39.15 | 9.9,37.5 9.9,38 9.28,38.62 9.26,38.62 | RN5.12 9.26,38.62 | RN5.13 9.27,37.5 9.9,37.5 | RN5.10 7.6,39.23 7.6,39.87 | RN5.11 v8.65,39.15 | v8.65,39.15 8.73,39.15 9.26,38.62 | RN4.8 11.75,45.11 11.75,44.4 11.95,44.2 | 12.5,43.65 11.95,44.2 | RN4.9 12.5,47.3 C2.2 | C17.2 4.8,46.44 U6.2 v4.8,50.4 4.75,50.45 C19.2 v4.75,53.55
  Bottom 0.3: v12.75,67.3 13.94,67.3
  Bottom 0.4: C24.2 15.65,18.1 14.75,17.2 13.73,17.2 13.1,16.57 C16.2
  Bottom 0.5: 13.47,14.13 J7.GND5 | 14.09,7.83 J7.6
  Bottom 0.55: 13.47,14.13 13.1,14.5 | J7.GND6 10.1,14.75 v10,14.85
  Bottom 0.6: J7.GND1 6.8,10.85 v6.8,11.8 J7.GND2 8.19,14.85 v8.6,14.85 v9.3,14.85 v10,14.85 v10.7,14.85 10.95,15.1 C16.2 13.1,14.5 | J7.GND4 J7.GND3 17.47,13.82 v17.65,14
  other vias: 3.2,15.7 5.15,21.1 5.15,20.5 10.05,18.55 10.05,19.15 3.9,6.5 22.2,12.65 15.5,46.65 15.9,56.6 15.9,55.55 15.95,54.2
  pour Top (no thermals): 10.85,28.63 10.85,29.97 10.9,30.02 11.15,30.02 11.22,29.95 11.22,28.63
  pour Route15 (isolate 0.3, rank 2): 0,0 22.9,0 22.9,68.6 0,68.6
  pour Route2 (isolate 0.3, rank 2): 0,0 22.9,0 22.9,68.6 0,68.6
  pour Bottom (no thermals): 10.65,32.9 12.15,32.9 12.3,32.75 12.3,32.1 11.15,30.95 10.8,30.95 10.5,31.25 10.5,32.75
  pour Bottom (no thermals): 3.8,12.8 3.8,17.25 3.61,17.44 3.61,19.19 3.2,19.6 3.2,20.45 3.35,20.6 4.25,20.6 4.4,20.45 4.4,19.65 4.85,19.65 5.5,20.3 5.5,21.2 5.3,21.4 3.85,21.4 3.7,21.55 3.7,22.3 3.4,22.3 3.4,21.7 2.9,21.2 2.9,19.5 3,19.4 3,17.4 3.2,17.2 3.2,16.05 2.95,15.8 2.2,15.8 2,16 1.3,16 1.25,15.95 1.25,15.45 1.3,15.4 2.4,15.4 3.2,14.6 3.2,12.85 3.25,12.8
  pour Bottom (no thermals): 7.2,16.65 7.2,17.4 9.3,19.5 10.25,19.5 10.5,19.25 10.5,17.55 10.68,17.37 12.03,17.37 12.1,17.3 12.1,16.88 12.04,16.82 10.93,16.82 10.85,16.9 7.76,16.9 7.47,16.61 7.24,16.61
GND_1
  cutout Route14 (rank 2): 11.45,30.05 11.22,30.27 12.85,31.9 13.25,31.5 15.25,31.5 18.62,28.12 14.68,24.18 11.45,27.4
GND_2
  cutout Route15 (rank 2): 11.45,30.05 11.22,30.27 12.85,31.9 13.25,31.5 15.25,31.5 18.62,28.12 14.68,24.18 11.45,27.4
GND_3
  cutout Route2 (rank 2): 11.45,30.05 11.22,30.27 12.85,31.9 13.25,31.5 15.25,31.5 18.62,28.12 14.68,24.18 11.45,27.4
GND_4
  cutout Route14 (rank 2): 9.18,31.93 10.82,30.27 10.6,30.05 10.6,27.7 7.35,24.45 3.35,28.45 6.4,31.5 8.75,31.5
GND_5
  cutout Route15 (rank 2): 9.18,31.93 10.82,30.27 10.6,30.05 10.6,27.7 7.35,24.45 3.35,28.45 6.4,31.5 8.75,31.5
GND_6
  cutout Route2 (rank 2): 9.18,31.93 10.82,30.27 10.6,30.05 10.6,27.7 7.35,24.45 3.35,28.45 6.4,31.5 8.75,31.5
GND_24  (via drill 0.2)
  Top 0.5: 11.85,29.45 11.85,28.92 SUPPLYTIE3.P$2 11.85,28.82 11.85,28.16
  other vias: 11.75,30.25 12.9,31.35 16.45,26.55 18,28.2 14.7,24.9 11.85,27.9 15.15,31.1
  pour Top (no thermals): 11.38,30.27 11.82,30.73 12.1,30.45 12.1,27.85 14.72,25.23 17.7,28.2 15,30.9 12.8,30.9 12.43,31.27 12.88,31.73 13.2,31.4 15.2,31.4 18.45,28.15 14.68,24.38 11.6,27.46 11.6,30.05
  pour Bottom (no thermals): 11.45,27.4 11.45,30.05 11.22,30.27 12.85,31.9 13.25,31.5 15.25,31.5 18.62,28.12 14.68,24.18
  cutout Route3 (rank 2): 11.45,30.05 11.22,30.27 12.85,31.9 13.25,31.5 15.25,31.5 18.62,28.12 14.68,24.18 11.45,27.4
GND_32  (via drill 0.2)
  Top 0.5: 10.23,29.6 10.23,28.9 SUPPLYTIE2.P$1 10.23,28.84 10.23,28.27
  other vias: 9.15,31.4 10.35,30.25 8.9,30 8.2,30 8.9,29.3 5.7,26.8 4,28.5 7.4,25.2 10.2,27.9 6.6,31.15
  pour Top (no thermals): 9.16,31.77 9.53,31.41 9.2,31.08 6.88,31.08 4.4,28.6 7.43,25.57 9.98,28.12 9.98,30.25 10.36,30.63 10.72,30.27 10.48,30.03 10.48,27.78 7.35,24.65 3.55,28.45 6.5,31.4 8.8,31.4
  pour Top (no thermals): 7.23,29.45 8.2,30.42 9.1,30.42 9.33,30.19 9.33,29.31 8.35,28.33
  pour Bottom (no thermals): 9.18,31.93 10.82,30.27 10.6,30.05 10.6,27.7 7.35,24.45 3.35,28.45 6.4,31.5 8.75,31.5
  cutout Route3 (rank 2): 9.18,31.93 10.82,30.27 10.6,30.05 10.6,27.7 7.35,24.45 3.35,28.45 6.4,31.5 8.75,31.5
GPIO0/!CS!/D0  (via drill 0.2)
  Top 0.15: v15.45,49.1 15.45,48.07 U1.55
  Route3 0.15: v11.05,43.3 11.35,43.6 11.6,43.6 15.45,47.45 v15.45,49.1
  Route14 0.15: J2.9 2.12,32.6 8.6,32.6 9.65,33.65 9.65,34.35 5.85,38.15 5.85,40.98 8.42,43.55 10.03,43.55 10.28,43.3 v11.05,43.3
GPIO1/D1  (via drill 0.2)
  Top 0.15: U1.7 8.43,33.87 v8.4,33.9
  Bottom 0.15: v8.4,33.9 8.4,33.52 7.29,32.41 6.06,32.41 5.62,31.97 3.59,31.97 J2.8
GPIO2/D2  (via drill 0.2)
  Top 0.15: U1.6 7.93,34.03 v7.82,34.14
  Bottom 0.15: J2.7 2.65,35.45 2.65,33.52 3.86,32.31 5.46,32.31 5.86,32.71 6.83,32.71 7.82,33.71 v7.82,34.14
GPIO3/D3  (via drill 0.2)
  Top 0.15: U1.5 7.43,33.91 v7.2,34.14
  Bottom 0.15: v7.2,34.14 7.18,34.12 7.18,33.77 6.41,33 5.55,33 5.2,32.65 4.17,32.65 3.1,33.72 3.1,36.81 2.62,37.29 2.62,38.02 J2.6
GPIO4/D4  (via drill 0.2)
  Top 0.15: U1.4 6.93,33.67 v6.6,34
  Route14 0.15: v6.6,34 | v6.6,34 6.17,33.57 5.72,33.57 5.47,33.82 5.47,35.73 4.35,36.85 3.7,36.85 3.2,37.35 3.2,39.98 J2.5
GPIO5/D5  (via drill 0.2)
  Top 0.15: U1.3 6.43,33.47 v5.9,34
  Route14 0.15: J2.4 2.22,44.45 2.52,44.15 2.83,44.15 3.2,43.78 3.2,40.72 3.44,40.48 3.44,37.91 3.75,37.6 4.35,37.6 5.9,36.05 v5.9,34
GPIO6/D6  (via drill 0.2)
  Top 0.15: v19.95,37.75 19.95,37.45 19.8,37.3 19.8,36.8 19.5,36.5 U1.30
  Route14 0.15: J2.3 2.73,48.45 11.4,48.45 17.3,42.55 17.85,42.55 18.9,41.5 18.9,40.3 19.8,39.4 19.8,38.75 19.95,38.6 v19.95,37.75
N$1
  Bottom 0.15: R9.1 3.1,12.1 2.6,12.1 2.24,12.46 2.24,12.92 1.88,13.28 1.42,13.28 0.9,13.8 0.9,19.8 1.49,20.39 CHG.2
N$2  (via drill 0.2)
  Top 0.15: v2.55,19.2 3.3,19.2 4.55,17.95 10.39,17.95 D5.A
  Bottom 0.15: v2.55,19.2 2.55,21.45 1.82,22.18 CHG.1
N$3  (via drill 0.2)
  Top 0.15: D5.C 10.4,17.6 4.35,17.6 4.25,17.7 v2.55,17.7
  Bottom 0.15: v2.55,17.7 U3.1
  Bottom 0.2: v2.55,17.7
N$4
  Bottom 0.15: R13.2 Q2.1
N$5
  Bottom 0.15: U3.5 2.09,14.11 R11.2
N$6  (via drill 0.2)
  Top 0.2: v1.3,59 1.3,59.88 D2.C
  Bottom 0.2: R5.2 v1.3,59
N$7  (via drill 0.2)
  Top 0.15: U1.92 5.45,38.5 6.75,39.8 8.4,39.8 8.95,40.35 8.95,40.8 8.6,41.15 8.25,41.15 7.6,41.8 7.6,42.35 6.65,43.3 v5.13,43.3
  Bottom 0.15: RN1.9 5.43,42.81 5.43,42.9 5.13,43.2 v5.13,43.3
N$8  (via drill 0.2)
  Top 0.15: v17.78,39.05 18.23,39.5 U1.36
  Bottom 0.15: RN3.9 17.18,38.46 v17.78,39.05
N$9  (via drill 0.2)
  Route3 0.12: v1.7,12.75 2.7,13.75 10.4,13.75 15.25,18.6 15.25,20.9 19.14,24.79 19.14,29.16 14.95,33.35 12.5,33.35 11.46,34.39 11.46,35.51 14.55,38.6 v14.55,39.85
  Bottom 0.15: R1.1 3,11.2 2.6,11.2 C1.2 2,11.7 1.7,12 v1.7,12.75 | RN3.7 14.58,39.85 v14.55,39.85
N$10
  Bottom 0.15: I2C.1 1.5,10.3 R6.2
N$11
  Bottom 0.15: I2C.3 1.5,6.5 R7.2
N$13  (via drill 0.2)
  Top 0.12: v13.3,35.65 13.93,35.02 U1.18
  Bottom 0.12: v13.3,35.65 14.25,35.65 RN3.14
N$14
  Bottom 0.2: R12.1 1.32,63.72 JP4.2
N$15  (via drill 0.2)
  Top 0.12: U1.25 17.43,33.61 v17.22,33.82 17.22,34.83 15.92,36.13 15.92,38.27 v16.6,38.95
  Bottom 0.12: v16.6,38.95 16.2,38.55 16.2,38.23 RN3.10 | v17.22,33.82 17.22,34.12 17.35,34.25 R2.2
N$16  (via drill 0.2)
  Top 0.2: D6.C 1.3,62.58 v1.3,61.65
  Bottom 0.2: v1.3,61.65 R12.2
N$17  (via drill 0.2)
  Top 0.15: U1.61 12.43,48.65 12.6,48.82 12.6,50 12.15,50.45 v12.15,51
  Bottom 0.15: RN1.14 7.8,46.1 7.8,46.79 9.78,48.77 9.78,49.88 10.9,51 v12.15,51
N$18  (via drill 0.2)
  Top 0.15: U1.60 12.93,50.32 v12.7,50.55
  Bottom 0.15: RN1.15 8.5,46.53 8.5,47.15 10.02,48.67 10.02,49.67 10.9,50.55 v12.7,50.55
N$19  (via drill 0.3)
  Top 0.3: J1.SHLD1 J1.SHLD6 J1.SHLD8 J1.SHLD2
  Bottom 0.3: J1.SHLD2 19.48,5.28 20.02,5.82 SHLD.2
  other vias: 7.11,5.28 15.75,5.28 15.75,1.1 7.11,1.1
N$20  (via drill 0.2)
  Top 0.15: J1.B5 13.18,5.41 12.75,4.98 12.75,3.97 13.17,3.55 v14.8,3.55 | v16.65,3.55 17.2,4.1 R3.2
  Bottom 0.15: v16.65,3.55 v14.8,3.55
N$21  (via drill 0.2)
  Top 0.15: R4.2 v6.25,3.95 | J1.A5 10.18,5.26 10.02,5.1 10.02,3.87 9.75,3.6 9.15,3.6 8.8,3.95 v8,3.95
  Bottom 0.15: v8,3.95 v6.25,3.95
N$22  (via drill 0.2)
  Top 0.15: U1.59 13.43,49.77 v13.4,49.8
  Bottom 0.15: v13.4,49.8 12.5,49.8 12.05,50.25 11.04,50.25 10.3,49.51 10.3,48.61 9.15,47.46 9.15,47.01 RN1.16
N$23  (via drill 0.2)
  Top 0.15: v17.62,43.89 v17.62,43.88 17.62,43.28 17.9,43 U1.43
  Bottom 0.15: RN4.15 17.32,43.89 v17.61,43.89 v17.62,43.89
N$24  (via drill 0.2)
  Top 0.15: U1.67 9.43,48.92 v9.35,49
  Bottom 0.15: RN1.13 7.35,45.42 7.35,47.05 9.3,49 v9.35,49
N$26  (via drill 0.2)
  Top 0.12: v13.75,36.1 14.2,35.65 14.2,35.28 14.43,35.05 U1.19
  Bottom 0.12: v13.75,36.1 13.85,36.1 14.05,36.3 14.73,36.3 RN3.13
N$27  (via drill 0.2)
  Top 0.12: v14.35,36.71 14.35,36.36 14.55,36.16 14.55,35.42 14.93,35.05 U1.20
  Bottom 0.12: RN3.12 15.34,36.83 14.62,36.83 14.5,36.71 v14.35,36.71
N$28  (via drill 0.2)
  Top 0.12: U1.21 15.43,35.02 14.9,35.55 v14.9,37.25
  Bottom 0.12: RN3.11 15.8,37.5 15.15,37.5 v14.9,37.25
N$29  (via drill 0.3)
  Top 0.2: U1.87 4.9,41 5.85,40.05 5.85,39.45 5.4,39 U1.91 v2.65,39
  Bottom 0.2: FB2.1 C27.1 C26.1 2.95,39.95 2.65,39.65 v2.65,39
N$30  (via drill 0.2)
  Top 0.15: U1.41 18.07,42 16.75,43.32 v16.75,44.75
  Bottom 0.15: v16.75,44.75 15.92,44.75 RN4.13
N$31  (via drill 0.2)
  Top 0.15: v17.3,45 17.3,45.3 17.7,45.7 18.13,45.7 18.33,45.5 U1.48
  Bottom 0.15: RN4.12 15.33,45.3 17,45.3 v17.3,45
N$32  (via drill 0.2)
  Top 0.15: U1.42 18.01,42.5 17.15,43.36 17.15,44.3 v17.2,44.35
  Bottom 0.15: v17.2,44.35 17.12,44.27 16.57,44.27 RN4.14
N$33  (via drill 0.3)
  Top 0.2: U1.8 8.93,32.25 8.6,31.92 v8.5,31.92
  Bottom 0.2: v8.5,31.92 6.19,31.92 3.12,28.86 3.12,28.12 7.05,24.2 BAT.2
N$35  (via drill 0.2)
  Top 0.15: U1.57 14.43,47.29 v14.22,47.08
  Bottom 0.15: v14.22,47.08 14.22,46.45 RN4.10
N$36  (via drill 0.2)
  Top 0.15: v14.95,46.05 14.93,46.07 U1.56
  Bottom 0.15: RN4.11 v14.95,46.05
N$37  (via drill 0.2)
  Top 0.15: U1.68 8.9,48.08 8.9,49.18 9.2,49.48 v9.2,49.9
  Bottom 0.15: RN1.12 6.9,44.73 6.9,47.16 9.2,49.46 v9.2,49.9
N$41  (via drill 0.2)
  Top 0.15: U1.93 4.83,38 v5.13,37.7
  Bottom 0.15: v5.13,37.7 5.62,38.19 RN5.8
N$42  (via drill 0.2)
  Top 0.15: U1.94 4.72,37.5 4.95,37.27 5.52,37.27 v5.55,37.3
  Bottom 0.15: v5.55,37.3 5.6,37.3 6.11,37.81 RN5.7
N$43  (via drill 0.2)
  Top 0.15: U1.95 5.24,37 5.39,36.85 v5.95,36.85
  Bottom 0.15: v5.95,36.85 6.35,36.85 RN5.6
N$44  (via drill 0.2)
  Top 0.15: U1.96 5.24,36.5 5.34,36.4 v6.35,36.4
  Bottom 0.15: v6.35,36.4 6.83,36.4 7.12,36.68 RN5.5
N$45  (via drill 0.2)
  Top 0.15: U1.97 6.15,36 6.2,35.95 v6.75,35.95
  Bottom 0.15: v6.75,35.95 7.72,35.95 RN5.4
N$46  (via drill 0.2)
  Top 0.15: U1.98 7.15,35.5 v7.2,35.45
  Bottom 0.15: v7.2,35.45 7.25,35.4 8.3,35.4 RN5.3
N$47
  Top 0.15: R15.2 Q1.1
N$97  (via drill 0.3)
  Top 0.2: v10.8,34.65 10.1,34.65 9.43,33.98 U1.9
  Bottom 0.2: C11.1 v10.8,34.65
N$98  (via drill 0.3)
  Top 0.2: v10.8,49.05 10.93,48.92 U1.64
  Bottom 0.2: v10.8,49.05 C12.1
QIO0  (via drill 0.2)
  Top 0.15: U1.73 6.42,49.21 7.16,49.95 7.85,49.95 12.7,54.8 16.15,54.8 16.75,55.4 16.75,56.7 16.25,57.2 15.45,57.2 v15.1,56.85
  Bottom 0.15: v15.1,56.85 14.65,56.85 14.5,56.7 U5.5
QIO1  (via drill 0.2)
  Top 0.15: U1.74 5.93,49.33 7.05,50.45 v7.4,50.45
  Bottom 0.15: U5.2 8.02,54.16 7.4,53.55 v7.4,50.45
QIO2  (via drill 0.2)
  Top 0.15: U1.71 7.43,49.03 v7.45,49.05
  Bottom 0.15: v7.45,49.05 6.85,49.65 6.85,54.65 7.63,55.44 U5.3
QIO3  (via drill 0.2)
  Top 0.15: U1.72 6.93,49.23 7.3,49.6 8.05,49.6 12.65,54.2 v15.1,54.2
  Bottom 0.15: v15.1,54.2 15.06,54.16 U5.7
QSPCLK  (via drill 0.2)
  Top 0.15: U1.75 5.43,49.48 7,51.05 8.3,51.05 12.75,55.5 v15.1,55.5
  Bottom 0.15: U5.6 15.04,55.44 v15.1,55.5
RA6_SWCLK/TCK  (via drill 0.2)
  Top 0.15: v19.6,47 19.18,47 18.98,46.8 U1.50
  Bottom 0.15: v19.6,47 19.6,48.97 J4.3
RA6_SWDIO/TMS  (via drill 0.2)
  Top 0.15: U1.51 17.43,49.42 v17.25,49.6
  Bottom 0.15: J4.2 17.25,51.32 v17.25,49.6
RA6_SWO/TDO/PICO/D18  (via drill 0.2)
  Top 0.15: v16.9,49.05 16.93,49.02 U1.52
  Bottom 0.15: J2.17 20.7,42.8 20.7,43.6 20.35,43.95 20.35,44.69 19.57,45.46 19.57,46.33 19.1,46.8 19.1,47.3 19.25,47.45 19.25,48.07 18.27,49.05 v16.9,49.05 15.75,50.2 15.75,50.28 J4.4
RA6_TDI/POCI/D17  (via drill 0.2)
  Top 0.15: U1.53 16.43,49.78 17.1,50.45 19.3,50.45 v19.75,50
  Bottom 0.15: J2.16 21.14,44.45 20.05,45.54 20.05,48.99 19.75,49.29 v19.75,50
RGB_DIN  (via drill 0.2)
  Top 0.15: U1.70 7.93,48.83 v8.15,49.05 | v2.2,59.1 2.2,63.94 D4.DI
  Route3 0.15: v8.15,49.05 8.15,50.85 8.7,51.4 8.7,53.2 2.8,59.1 v2.2,59.1
RGB_DOUT  (via drill 0.2)
  Top 0.15: D4.DO 3.54,67.3 v3.55,67.3
  Bottom 0.15: TP1.1 | v3.55,67.3 TP1.1
RX_RA6/TX_DA14531  (via drill 0.2)
  Top 0.15: v5.7,59.55 5.68,59.57 U2.5 | U1.66 9.93,50.22 v9.7,50.45
  Route3 0.15: v9.7,50.45 9.7,55.55 v5.7,59.55
  Bottom 0.15: v5.7,59.55 5.7,60.31 TP6.1
SCK/D19  (via drill 0.2)
  Top 0.15: J2.18 20.73,40.23 20.73,40.83 20.3,41.26 20.3,42.22 20.55,42.47 20.55,43.53 20.36,43.72 20.36,45.12 v20.85,45.6 | v19.2,51.3 17.05,51.3 15.93,50.18 U1.54
  Bottom 0.15: v20.85,45.6 20.35,46.1 20.35,49.13 20.2,49.28 20.2,50.3 v19.2,51.3
SCL/D16  (via drill 0.2)
  Top 0.15: J3.4 v3.9,7.4 3.2,7.4 2,8.6 2,9.54 4.13,11.67 4.13,15.57 3.35,16.35 1.81,16.35 1.2,16.96 1.2,19.09 2.16,20.05 3.8,20.05 4.05,20.3 v4.05,23 | v3.9,31.25 4.55,31.25 5.43,32.13 U1.1
  Route3 0.15: J2.2 3.85,46.95 3.85,31.65 3.9,31.6 v3.9,31.25
  Bottom 0.15: R7.1 3.4,7.4 v3.9,7.4 | U7.7 v4.05,23 4.05,26.25 2.5,27.8 2.5,29.86 v3.9,31.25
SDA/D15  (via drill 0.2)
  Top 0.15: J3.3 v3.9,8.4 2.8,8.4 2.45,8.75 2.45,9.35 4.58,11.48 4.58,15.76 3.54,16.8 2,16.8 1.65,17.15 1.65,18.95 2.35,19.65 4.04,19.65 4.55,20.16 v4.55,22.7 | U1.2 5.93,32.08 4.67,30.82 v4.33,30.82
  Route3 0.15: J2.1 4.18,49.16 4.18,31.82 4.33,31.67 v4.33,30.82
  Bottom 0.15: v3.9,8.4 3.9,9.3 2.5,10.7 R6.1 | U7.8 v4.55,22.7 4.55,26.15 2.75,27.95 2.75,29.23 v4.33,30.82
SDCLK  (via drill 0.2)
  Top 0.12: v18.1,37.75 18.1,37.77 18.33,38 U1.33
  Bottom 0.12: v18.1,37.75 18.1,36.93 15.29,34.12 15.29,33.67 19.97,28.99 19.97,26.12 18.8,24.95 18.8,8.4 18.35,7.95 15.35,7.95 14.9,8.4 13.4,8.4 12.99,7.99 J7.5
SDCMD  (via drill 0.2)
  Top 0.12: U1.34 v18.05,38.5
  Bottom 0.12: v18.05,38.5 18.05,38.31 17.64,37.9 17.64,37.6 17.76,37.47 17.76,36.94 15.03,34.21 15.03,33.63 19.76,28.9 19.76,26.56 18.25,25.05 18.25,8.4 18.1,8.24 15.51,8.24 15.1,8.65 11.35,8.65 10.79,8.09 J7.3
SDDAT0  (via drill 0.2)
  Top 0.12: v19.85,40 U1.37
  Bottom 0.12: v19.85,40 18.65,38.8 18.65,37.19 15.55,34.09 15.55,33.7 20.18,29.07 20.18,25.63 19.35,24.8 19.35,8.4 18.59,7.64 15.34,7.64 15.19,7.49 J7.7
SDDAT1  (via drill 0.2)
  Top 0.12: U1.22 15.93,33.58 16.01,33.66 v16.01,33.86
  Bottom 0.12: v16.01,33.86 16.06,33.81 16.06,33.54 20.39,29.21 20.39,25.14 19.9,24.65 19.9,8.4 18.83,7.33 17.23,7.33 16.79,6.89 J7.8
SDDAT2  (via drill 0.2)
  Top 0.12: U1.31 18.33,37 18.18,36.85 17.15,36.85 17,37 v16.85,37
  Bottom 0.12: v16.85,37 16.6,36.75 16.6,36.47 14.51,34.38 14.51,33.55 19.34,28.73 19.34,27.55 17.15,25.36 17.15,14.9 15.75,13.5 8,13.5 7.58,13.08 7.58,8.57 8.59,7.56 J7.1
SDDAT3  (via drill 0.2)
  Top 0.12: U1.32 18.55,37.5 18.35,37.3 v17.35,37.3
  Bottom 0.12: v17.35,37.3 17.35,36.88 14.77,34.3 14.77,33.59 19.55,28.81 19.55,27.03 17.75,25.23 17.75,14.91 15.89,13.05 8.33,13.05 7.98,12.7 7.98,8.72 8.35,8.35 9.2,8.35 9.69,7.86 J7.2
SDDET  (via drill 0.2)
  Top 0.12: v20.28,38.9 19.73,38.9 19.63,39 U1.35
  Route3 0.15: v6.65,7.5 14.05,14.9 14.05,15.6 20,21.55 20,30.35 v18.85,31.5
  Bottom 0.12: v20.28,38.9 20.28,38.05 20.43,37.9 20.43,36.38 20.79,36.02 20.79,35.28 20.2,34.69 20.2,32.85 v18.85,31.5
  Bottom 0.2: J7.9 6.84,9.52 6.84,8.49 6.65,8.3 v6.65,7.5
STAT_LED  (via drill 0.2)
  Top 0.15: U1.69 8.45,48.07 8.45,48.73 8.65,48.93 v8.65,49.55 | D2.A 3.65,59.33 v3.65,59
  Route3 0.15: v8.65,49.55 8.65,50.75 9.25,51.35 9.25,54 4.25,59 v3.65,59
TX_RA6/RX_DA14531  (via drill 0.2)
  Top 0.15: v19.25,63.7 17.2,63.7 U2.14 | U1.65 10.43,48.69 10.3,48.82 v10.3,51.1
  Route3 0.2: v19.25,63.7 12.75,63.7 10.3,61.25 v10.3,51.1
  Bottom 0.15: TP5.1 v19.25,63.7
UART_RX/D21  (via drill 0.2)
  Top 0.15: U1.24 16.93,33.45 16.78,33.6 16.78,34.67 15.65,35.8 15.65,44.4 v17.05,45.8
  Route14 0.15: v17.05,45.8 20.4,45.8 J2.15
UART_TX/D20  (via drill 0.2)
  Top 0.15: U1.23 16.43,33.42 16.44,33.43 16.44,34.51 15.35,35.6 15.35,44.8 v16.35,45.8
  Route14 0.15: J2.14 19.69,47.63 18.18,47.63 v16.35,45.8
USBD_N
  Top 0.16: D1.4 11.93,9.58 12.13,9.78 12.13,10.53 11.62,11.04 11.62,11.47 12.3,12.15 18.26,12.15 19.88,13.77 19.88,32.55 18.13,34.3 18.13,34.7 18.43,35 U1.27
USBD_P
  Top 0.16: D1.6 10.93,9.58 10.73,9.78 10.73,10.53 11.24,11.04 11.24,11.63 12.14,12.53 18.1,12.53 19.5,13.93 19.5,32.4 17.75,34.15 17.75,34.86 18.39,35.5 U1.28
USBIN_N  (via drill 0.2)
  Top 0.16: J1.B7 10.68,5.21 10.63,5.16 v10.63,4.8 | v11.73,4.8 11.73,5.21 11.68,5.26 J1.A7 11.68,7.18 12.03,7.53 12.03,8.22 11.93,8.32 D1.3
  Bottom 0.16: v11.73,4.8 v10.63,4.8
USBIN_P
  Top 0.16: J1.B6 12.18,5.16 12.28,5.06 12.28,4.58 11.97,4.27 11.48,4.27 11.18,4.57 11.18,5.21 J1.A6 11.18,7.17 10.83,7.52 10.83,8.24 10.93,8.35 D1.1
V_BATT  (via drill 0.3)
  Top 0.5: J2.12 4.12,24.13 6.05,22.2 v6.05,19.7
  other vias: 6.85,19.7 7.65,19.7 8.45,19.7
  pour Bottom (isolate 0.15, rank 2, no thermals): 4.14,20.36 3.46,20.36 3.4,20.3 3.4,19.7 4,19.1 4,17.45 4.2,17.25 4.2,16.15 4.7,16.15 4.7,17.1 5.1,17.5 6.55,17.5 6.7,17.35 6.7,16.65 7,16.65 7,17.6 8.9,19.5 8.9,19.9 8.75,20.05 5.75,20.05 5,19.3 4.45,19.3 4.2,19.55 4.2,20.3
  pour Top (isolate 0.15, rank 2, no thermals): 4.95,19.45 5.8,20.3 6.3,20.3 6.55,20.05 8.75,20.05 9.55,19.25 9.55,18.3 5,18.3 4.95,18.35
V_USB  (via drill 0.3)
  Top 0.25: v11.43,10.25 D1.5
  Top 0.6: v5.95,14.6 7,15.65 11.75,15.65 12.35,16.25 12.35,19.65 10.35,21.65 8.93,21.65 1.37,29.21 J2.10
  Route3 0.25: v13.45,4.85 13.38,4.85 12.73,5.5 12.73,8.95 v11.43,10.25
  other vias: 9.45,4.25 9.45,4.85 13.45,4.25
  pour Top (isolate 0.15, rank 2, no thermals): 9.27,6.3 9.27,5.33 9.45,5.15 9.6,5.15 9.9,4.85 9.9,4 9.65,3.75 9.25,3.75 9.05,3.95 9.05,4.95 8.7,5.3 8.7,6.3
  pour Top (isolate 0.15, rank 2, no thermals): 13.6,6.35 13.6,5.3 13.45,5.15 13.25,5.15 13.1,5 13.1,4.1 13.28,3.92 13.57,3.92 13.8,4.15 13.8,4.95 14.15,5.3 14.15,6.35
  pour Bottom (isolate 0.15, rank 2, no thermals): 9.05,4.95 9.25,5.15 9.6,5.15 10.55,4.2 11.75,4.2 12.7,5.15 13.6,5.15 13.8,4.95 13.8,4.2 11.7,2.1 5.3,2.1 4.4,3 4.4,8.65 4.15,8.9 4.15,14.65 4.4,14.9 6.55,14.9 6.7,15.05 6.7,15.75 7,15.75 7,14.55 6.85,14.4 6.25,14.4 5.75,13.9 5.75,3.8 6.05,3.5 8.3,3.5 9.05,4.25
VIN  (via drill 0.3)
  Route3 0.2: v11.45,42.35 11.45,37.5 10,36.05 10,34.3 11.45,32.85 14.79,32.85 18.78,28.86 18.78,25.63 v13.3,20.15
  Route14 0.2: v6.1,44.45 6.7,45.05 10.5,45.05 12,43.55 12,42.9 v11.45,42.35
  Bottom 0.2: U6.1 5.75,46.91 | C17.1 5.85,46.35 6.1,46.11 v6.1,44.45 | v13.3,20.15 R10.2
  Bottom 0.3: 5.75,46.91 C17.1
  Bottom 0.35: R10.2 13.3,18.7 12.5,17.9 12.5,16.7 11.95,16.15 U4.1
  pour Bottom (isolate 0.15, rank 2, no thermals): 6.45,17.25 6.25,17.25 6.2,17.2 6.2,15.2 6.25,15.15 6.45,15.15 6.5,15.2 6.5,15.85 6.65,16 7.55,16 7.75,15.8 10.9,15.8 11,15.9 12.05,15.9 12.1,15.95 12.1,16.3 12,16.4 10.95,16.4 10.75,16.6 7.75,16.6 7.55,16.4 6.65,16.4 6.5,16.55 6.5,17.2
VREF1  (via drill 0.3)
  Route3 0.2: v5.75,54.05 5.75,45.7 9.25,42.2 9.25,33.85 8.7,33.3 v4.8,33.3 4.86,33.24 4.86,30.56 3.25,28.95 3.25,28 7.9,23.35 v8.9,23.35
  Route14 0.2: J2.26 13.2,19.05 v8.9,23.35
  Bottom 0.2: U6.5 C19.1 v5.75,54.05 | FB2.2 4.4,37.2 4.8,36.8 v4.8,33.3
VREFEN  (via drill 0.2)
  Top 0.15: v8.55,41.95 8.55,43.8 5.85,46.5 U1.76
  Top 0.2: U1.76 3.13,46.5 2.93,46.7 v2.9,46.7
  Bottom 0.2: U6.3 3.85,45.76 TP2.1 3.81,45.79 v2.9,46.7 | RN1.6 v8.55,41.95
VREG_EN  (via drill 0.2)
  Route3 0.15: J2.11 2.5,25.44 2.5,20.4 3.9,19 8.9,19 9.65,19.75 v11.1,19.75
  Bottom 0.15: R10.1 11.75,19.75 v11.1,19.75
  Bottom 0.2: U4.3 11.85,18.05 12.3,18.5 R10.1
XCIN
  Top 0.15: U1.10 9.93,31.28 9.35,30.7 7.49,30.7 C10.2 6.65,29.85 6.65,29.51 Y2.P$1
XCOUT
  Top 0.15: U1.11 10.43,31.23 9.6,30.4 9.6,28.59 C9.2 8.75,27.75 8.41,27.75 Y2.P$2
XTAL
  Top 0.15: U1.13 11.43,31.43 14.89,27.97 14.89,26.66 Y1.3

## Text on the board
Top: 1
Route2: 2
Route3: 3
Route14: 4
Route15: 5
Bottom: 6 | v10
Measures: All Units in Inches
tDocu: Layers: 6 / Stackup: JLC06161H-3313 / Material: TG155 / Outer Layers: 1oz / Inner Layers: 0.5oz / Board thickness: 1.6mm / Via Covering: Epoxy Filled & Capped / Soldermask: Red / Silkscreen: White / Surface Finish: ENIG | Alex Brudner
